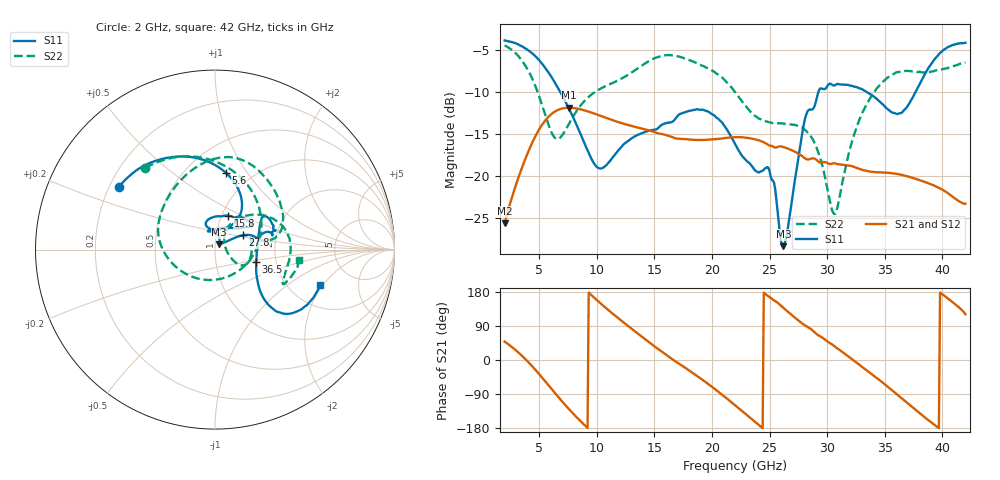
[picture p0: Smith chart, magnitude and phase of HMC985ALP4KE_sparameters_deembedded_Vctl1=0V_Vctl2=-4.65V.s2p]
!s2p File: Measurements: S11, S21, S12, S22
# GHz S dB R 50.0
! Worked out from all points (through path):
!   401 points, 2 GHz to 42 GHz, reference 50 ohm
!   highest |S21| = -11.89 dB at 7.6 GHz (marker M1); lowest = -25.7 dB at 2 GHz (marker M2)
!   lowest |S11| = -28.4 dB at 26.2 GHz (marker M3), VSWR 1.08, Z = 52.3 + j3.17 ohm
!   |S11| at or under -10 dB: 6.82 GHz to 29.25 GHz (22.43 GHz wide, 124 % of centre); 33.42 GHz to 37.69 GHz (4.267 GHz wide, 12 % of centre)
!   |S22| runs from -24.5 to -4.5 dB; largest |S21 - S12| = 0.00021
!   S11 on the Smith chart (normalised r, x): 2 GHz: 0.24, +0.28; 5.6 GHz: 0.76, +0.80; 15.8 GHz: 1.07, +0.42; 27.8 GHz: 1.34, +0.22; 36.5 GHz: 1.57, -0.23; 42 GHz: 2.94, -1.89
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2  -3.88 147.0  -25.66 48.6  -25.67 48.6  -4.47 130.5
3.6  -4.66 120.3  -18.70 8.4  -18.70 8.4  -6.47 84.9
4.7  -5.80 99.5  -15.22 -26.8  -15.22 -26.8  -9.41 43.4
5.6  -7.29 81.9  -13.29 -59.0  -13.30 -59.0  -13.04 -3.7
6.5  -9.22 66.5  -12.25 -91.9  -12.25 -92.0  -15.60 -68.8
7.6  -12.04 54.8  -11.89 -130.1  -11.90 -130.1  -13.77 -135.7
8.7  -15.38 55.1  -12.12 -164.7  -12.12 -164.7  -11.45 -170.2
10.4  -19.12 89.6  -12.90 147.6  -12.90 147.5  -9.57 162.5
15.4  -14.23 75.7  -14.97 27.6  -14.97 27.6  -5.81 87.2
15.8  -13.83 68.7  -15.07 18.7  -15.07 18.6  -5.67 82.1
19.4  -12.23 33.3  -15.72 -57.2  -15.73 -57.2  -7.04 35.1
22  -16.18 51.1  -15.40 -119.3  -15.41 -119.3  -10.02 9.8
24.9  -19.04 104.8  -16.34 168.0  -16.34 168.0  -13.59 13.2
26.2  -28.39 52.8  -16.57 137.6  -16.57 137.6  -13.79 -2.3
27.8  -15.23 27.2  -17.63 97.1  -17.63 97.1  -14.23 -24.2
28.7  -12.10 12.6  -17.93 79.0  -17.93 79.0  -15.53 -31.3
30.7  -9.21 20.8  -18.53 34.7  -18.53 34.7  -24.54 21.9
32.8  -9.59 33.9  -19.18 -12.9  -19.18 -12.9  -13.30 53.5
35.4  -12.21 11.8  -19.66 -74.1  -19.66 -74.1  -8.18 21.6
36.5  -12.48 -16.6  -19.91 -101.9  -19.90 -101.9  -7.53 7.5
39.5  -5.85 -43.7  -21.31 -175.2  -21.32 -175.4  -7.44 -26.4
42  -4.16 -18.6  -23.34 120.7  -23.33 120.6  -6.48 -7.3
